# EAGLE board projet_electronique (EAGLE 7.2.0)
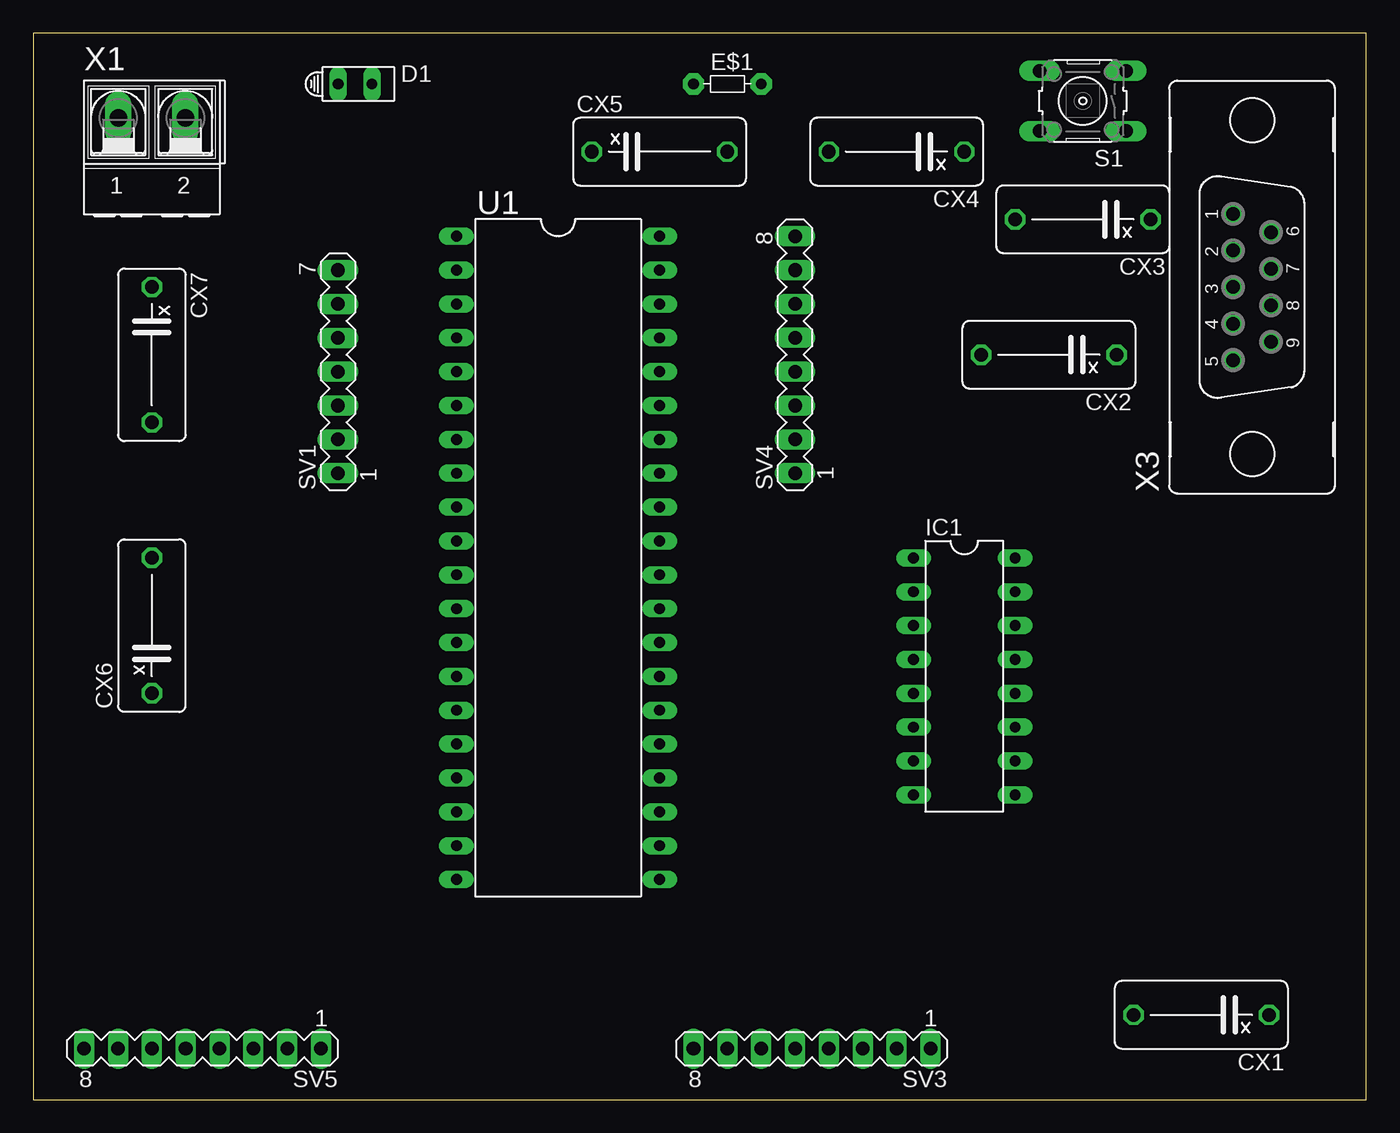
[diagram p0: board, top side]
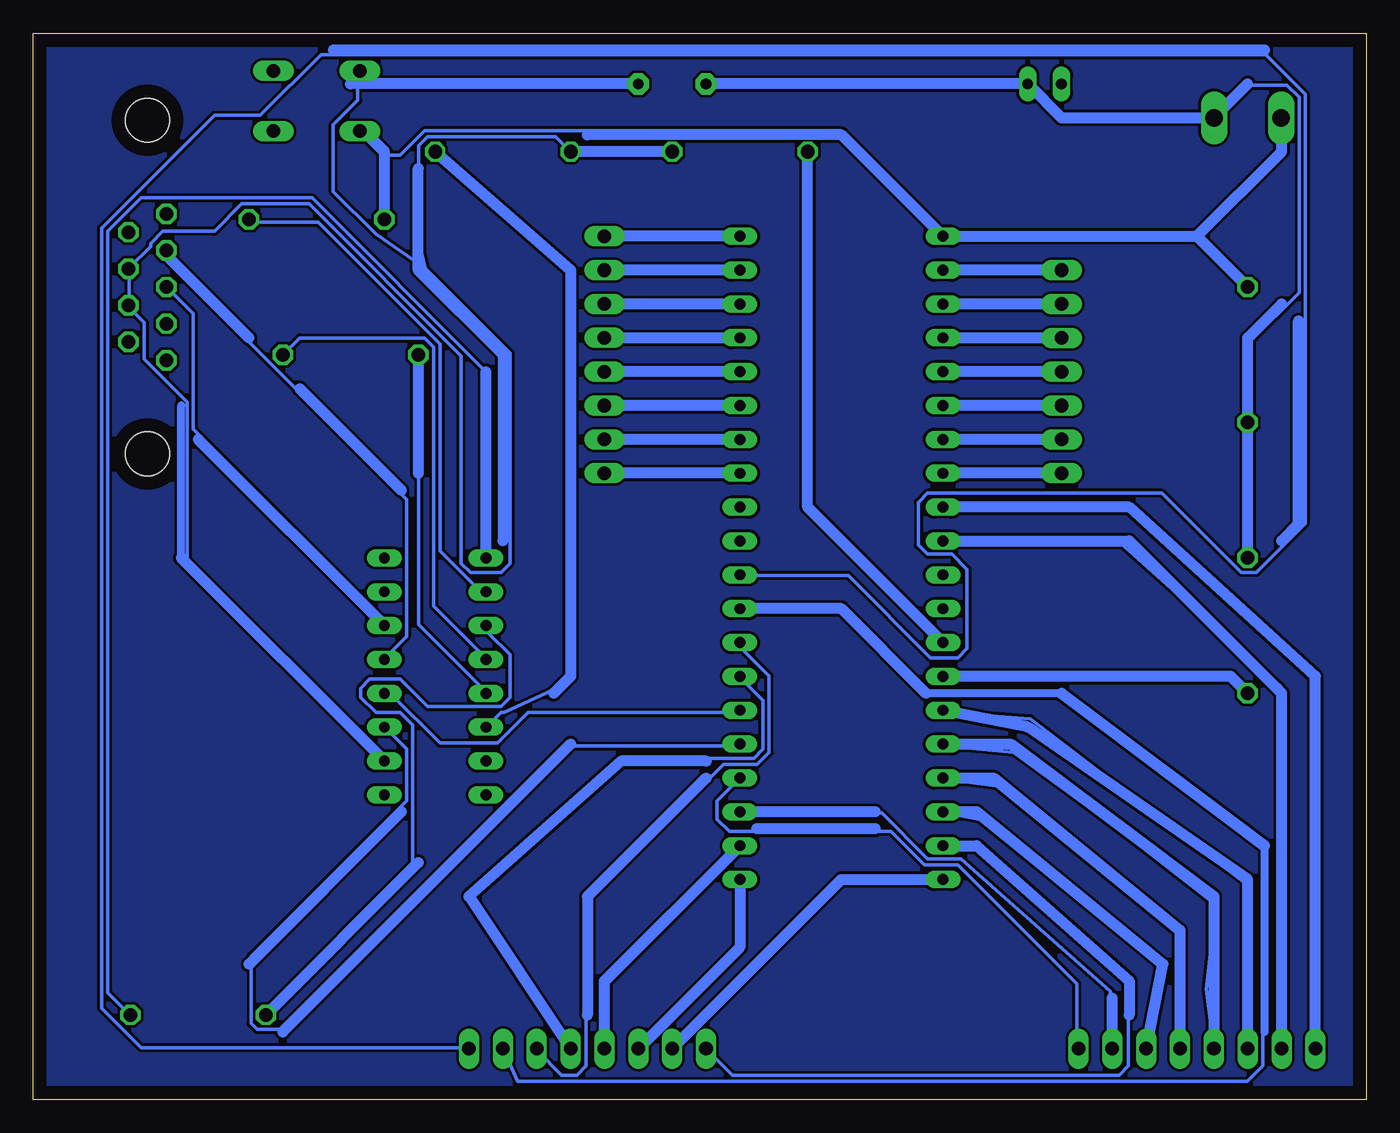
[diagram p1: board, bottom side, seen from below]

Size 100 x 80 mm. Coordinates in mm from the lower left corner, seen from the top.
Outline: 0,0 100,0 100,80 0,80 0,0
Copper layers (1*16): Top 0.035mm / dielectric 1.5mm / Bottom 0.035mm
Design rules "default": minimum track width 10mil, minimum drill 24mil, track to track 8mil, track to pad 8mil, pad to pad 8mil, via to via 8mil, smd to smd 8mil, copper to edge 40mil, drill to drill 8mil, minimum pad ring 10mil, minimum via ring 8mil, stop-mask expansion 4mil, vias tented up to drill 0mil, thermal gap 10mil

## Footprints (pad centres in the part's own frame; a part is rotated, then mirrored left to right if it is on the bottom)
XC10B5 = drill 1.016 octagon: 1 -5.08,0; 2 5.08,0
HLMP6 = drill 0.813 long: A -1.27,0; K 1.27,0
R-5 = drill 0.813 pad 1.6 octagon: 1 -2.54,0; 2 2.54,0
DIL16 = drill 0.813 long: 1 -8.89,-3.81; 2 -6.35,-3.81; 3 -3.81,-3.81; 4 -1.27,-3.81; 5 1.27,-3.81; 6 3.81,-3.81; 7 6.35,-3.81; 8 8.89,-3.81; 9 8.89,3.81; 10 6.35,3.81; 11 3.81,3.81; 12 1.27,3.81; 13 -1.27,3.81; 14 -3.81,3.81; 15 -6.35,3.81; 16 -8.89,3.81
B3F-10XX = drill 1.016 long: 1 -3.251,2.261; 2 3.251,2.261; 3 -3.251,-2.261; 4 3.251,-2.261
MA07-1 = drill 1.016 long: 1 -7.62,0; 2 -5.08,0; 3 -2.54,0; 4 0,0; 5 2.54,0; 6 5.08,0; 7 7.62,0
MA08-1 = drill 1.016 long: 1 -8.89,0; 2 -6.35,0; 3 -3.81,0; 4 -1.27,0; 5 1.27,0; 6 3.81,0; 7 6.35,0; 8 8.89,0
DIL40 = drill 0.813 long: 1 -24.13,-7.62; 2 -21.59,-7.62; 3 -19.05,-7.62; 4 -16.51,-7.62; 5 -13.97,-7.62; 6 -11.43,-7.62; 7 -8.89,-7.62; 8 -6.35,-7.62; 9 -3.81,-7.62; 10 -1.27,-7.62; 11 1.27,-7.62; 12 3.81,-7.62; 13 6.35,-7.62; 14 8.89,-7.62; 15 11.43,-7.62; 16 13.97,-7.62; 17 16.51,-7.62; 18 19.05,-7.62; 19 21.59,-7.62; 20 24.13,-7.62; 21 24.13,7.62; 22 21.59,7.62; 23 19.05,7.62; 24 16.51,7.62; 25 13.97,7.62; 26 11.43,7.62; 27 8.89,7.62; 28 6.35,7.62; 29 3.81,7.62; 30 1.27,7.62; 31 -1.27,7.62; 32 -3.81,7.62; 33 -6.35,7.62; 34 -8.89,7.62; 35 -11.43,7.62; 36 -13.97,7.62; 37 -16.51,7.62; 38 -19.05,7.62; 39 -21.59,7.62; 40 -24.13,7.62
AK500/2-H = drill 1.321 long: 1 -2.515,0; 2 2.515,0
F09V = drill 1.016 octagon: 1 5.486,1.422; 2 2.743,1.422; 3 0,1.422; 4 -2.743,1.422; 5 -5.486,1.422; 6 4.115,-1.422; 7 1.372,-1.422; 8 -1.372,-1.422; 9 -4.115,-1.422 | hole 3.302: -12.522,0; 12.522,0

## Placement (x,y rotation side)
CX1  1u  [XC10B5]  87.63,6.35 180 top
CX2  1u  [XC10B5]  76.2,55.88 180 top
CX3  1u  [XC10B5]  78.74,66.04 180 top
CX4  1u  [XC10B5]  64.77,71.12 180 top
CX5  15p  [XC10B5]  46.99,71.12 0 top
CX6  15p  [XC10B5]  8.89,35.56 90 top
CX7  680n  [XC10B5]  8.89,55.88 270 top
D1  HLMP6  [HLMP6]  24.13,76.2 0 top
E$1  [R-5]  52.07,76.2 0 top
IC1  MAX232  [DIL16]  69.85,31.75 270 top
S1  [B3F-10XX]  78.74,74.93 180 top
SV1  [MA07-1]  22.86,54.61 90 top
SV3  [MA08-1]  58.42,3.81 180 top
SV4  [MA08-1]  57.15,55.88 90 top
SV5  [MA08-1]  12.7,3.81 180 top
U1  PIC16F877P  [DIL40]  39.37,40.64 270 top
X1  [AK500/2-H]  8.89,73.66 0 top
X3  [F09V]  91.44,60.96 90 top

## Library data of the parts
CX1-CX7 = rcl
D1 = display-hp; MF: AGILENT TECHNOLOGIES; MPN: HLMP-6500; OC_FARNELL: 1652490; OC_NEWARK: 40K0088
E$1 = discrete
IC1 = maxim; MF: MAXIM; MPN: MAX232ACPE+; OC_FARNELL: 9723773; OC_NEWARK: 68K4544
S1 = switch-omron; MPN: B3F-1000; OC_FARNELL: 176432; OC_NEWARK: 36M3542
SV1 SV3-SV5 = con-lstb; OC_FARNELL: unknown; OC_NEWARK: unknown
U1 = pic16f87x
X1 = con-ptr500; OC_FARNELL: unknown; OC_NEWARK: unknown
X3 = con-subd; OC_FARNELL: unknown; OC_NEWARK: unknown

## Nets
GND: IC1.15
N$1: D1.A
N$2: CX3.2 CX7.1 S1.2 U1.1 X1.1
N$3: CX4.2 CX5.2 IC1.10 S1.4 X3.7 X3.8
N$4: CX5.1 U1.13
N$5: CX1.1 IC1.1
N$7: CX6.1 U1.14
N$8: CX1.2 IC1.3
N$9: CX2.1 IC1.4
N$10: CX2.2 IC1.5
N$11: CX3.1 IC1.2
N$12: CX4.1 IC1.6
N$13: IC1.11 U1.25
N$14: IC1.12 U1.26
N$15: SV1.7 U1.2
N$16: IC1.14 X3.3
N$17: IC1.13 X3.2
N$18: SV4.1 U1.33
N$19: SV4.2 U1.34
N$20: SV4.3 U1.35
N$21: SV4.4 U1.36
N$22: SV1.6 U1.3
N$23: SV1.5 U1.4
N$24: SV1.4 U1.5
N$25: SV1.3 U1.6
N$26: SV1.2 U1.7
N$27: SV1.1 U1.8
N$28: SV3.8 U1.19
N$29: SV3.7 U1.20
N$30: SV3.6 U1.21
N$31: SV3.5 U1.22
N$32: SV3.4 U1.27
N$33: SV3.3 U1.28
N$34: SV3.2 U1.29
N$35: SV3.1 U1.30
N$36: SV4.5 U1.37
N$37: SV4.6 U1.38
N$38: SV4.7 U1.39
N$39: SV4.8 U1.40
N$40: SV5.8 U1.9
N$41: SV5.7 U1.10
N$42: SV5.6 U1.15
N$43: SV5.5 U1.16
N$44: SV5.4 U1.17
N$45: SV5.3 U1.18
N$46: SV5.2 U1.23
N$47: SV5.1 U1.24
S$1: CX6.2 CX7.2 D1.K E$1.1 X1.2
S$2: E$1.2
VCC: IC1.16

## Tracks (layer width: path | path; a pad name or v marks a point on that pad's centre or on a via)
N$2
  Bottom 0.254: 73.84,70.87 73.84,66.06 CX3.2 | 73.84,70.87 75.44,72.47 S1.2 | 12.57,64.69 31.55,64.69 U1.1 31.77,64.92 39.55,72.69 70.64,72.69 72.47,70.87 73.84,70.87 | 12.57,64.69 8.91,61.04 CX7.1 | 12.57,64.69 6.4,70.87 6.4,73.61 X1.1
  Bottom 0.813: 12.7,64.77 U1.1 39.37,72.39 58.42,72.39 | 12.7,64.77 CX7.1 | 12.7,64.77 6.35,71.12 6.35,73.66 | CX3.2 73.66,71.12 74.93,72.39
N$3
  Bottom 0.254: IC1.10 73.84,25.6 88.47,40.23 88.47,52.35 91.67,55.55 91.67,58.29 92.81,59.44 X3.8 92.81,59.66 92.81,62.18 X3.7 92.81,62.41 91.21,64.01 91.21,64.24 90.3,65.15 86.41,65.15 84.35,67.21 79.32,67.21 67.89,55.78 67.89,40.23 67.21,39.55 64.92,39.55 64.24,40.23 64.24,56.01 70.61,62.38 | CX5.2 52.12,71.09 59.66,71.09 CX4.2 60.81,72.24 70.41,72.24 71.09,71.55 71.09,64.44 70.61,62.38 | 70.61,62.38 74.3,64.92 77.5,68.12 77.5,73.15 75.67,74.98 75.67,77.04 S1.4
  Bottom 0.61: 88.9,40.64 88.9,52.07
  Bottom 0.813: CX5.2 CX4.2 | IC1.10 88.9,40.64
N$4
  Bottom 0.254: U1.13 31.77,34.29 31.77,34.75 41.83,44.81 41.83,71.09 CX5.1
  Bottom 0.813: U1.13 41.91,44.45 CX5.1
N$5
  Bottom 0.254: IC1.1 66.06,40.69 66.06,54.63 79.1,67.67 91.9,67.67 94.41,65.15 94.41,8 92.81,6.4 CX1.1
  Bottom 0.813: IC1.1 66.04,54.61
N$7
  Bottom 0.254: U1.14 31.55,31.55 9.83,31.55 8.91,30.63 CX6.1
  Bottom 0.813: CX6.1 10.16,31.75 U1.14
N$8
  Bottom 0.254: IC1.3 65.84,35.43 65.84,34.98 64.24,33.38 64.24,30.18 64.92,29.49 70.41,29.49 72.47,31.55 74.75,31.55 75.44,30.86 75.44,30.18 74.3,29.03 72.47,29.03 71.55,28.12 71.55,17.37 82.53,6.4 CX1.2
  Bottom 0.813: CX1.2 71.12,17.78
N$9
  Bottom 0.254: CX2.1 80.01,57.15 70.64,57.15 69.95,56.46 69.95,37.03 66.06,33.15 IC1.4
N$10
  Bottom 0.254: IC1.5 66.06,30.63 71.09,35.66 71.09,55.78 CX2.2
  Bottom 0.813: CX2.2 71.12,46.99
N$11
  Bottom 0.254: IC1.2 66.06,38.18 66.52,38.18 69.49,41.15 69.49,56.69 78.64,65.84 83.67,65.84 CX3.1
N$12
  Bottom 0.254: IC1.6 65.84,28.12 64.92,29.03 64.69,29.03 59.97,31.22 59.97,62.61 69.72,71.09 CX4.1
  Bottom 0.813: CX4.1 59.69,62.23 59.69,31.75 60.96,30.48
N$13
  Bottom 0.254: IC1.11 72.01,26.29 72.01,22.4 83.67,10.74 83.67,5.71 83.21,5.26 81.38,5.26 60.12,26.52 47.09,26.52 U1.25
N$14
  Bottom 0.254: U1.26 47.09,29.03 62.87,29.03 65.15,26.75 69.49,26.75 73.15,30.4 73.61,30.4 IC1.12
N$15
  Bottom 0.254: U1.2 31.55,62.41 22.86,62.41 SV1.7
  Bottom 0.813: SV1.7 U1.2
N$16
  Bottom 0.254: IC1.14 73.84,35.66 73.84,36.12 88.01,50.29 88.01,58.98 89.84,60.81 X3.3
  Bottom 0.813: IC1.14 87.63,49.53
N$17
  Bottom 0.254: IC1.13 73.61,33.15 72.01,34.75 72.01,45.03 89.84,62.87 89.84,63.55 X3.2
N$18
  Bottom 0.254: U1.33 47.09,47.09 57.15,47.09 SV4.1
  Bottom 0.813: U1.33 SV4.1
N$19
  Bottom 0.254: U1.34 47.09,49.61 57.15,49.61 SV4.2
  Bottom 0.813: U1.34 SV4.2
N$20
  Bottom 0.254: U1.35 47.09,52.12 57.15,52.12 SV4.3
  Bottom 0.813: U1.35 SV4.3
N$21
  Bottom 0.254: U1.36 47.09,54.63 57.15,54.63 SV4.4
  Bottom 0.813: U1.36 SV4.4
N$22
  Bottom 0.254: U1.3 31.55,59.89 22.86,59.89 SV1.6
  Bottom 0.813: SV1.6 U1.3
N$23
  Bottom 0.813: SV1.5 U1.4
N$24
  Bottom 0.254: U1.5 31.55,54.63 22.86,54.63 SV1.4
  Bottom 0.813: SV1.4 U1.5
N$25
  Bottom 0.254: U1.6 31.55,52.12 22.86,52.12 SV1.3
  Bottom 0.813: SV1.3 U1.6
N$26
  Bottom 0.254: U1.7 31.55,49.61 22.86,49.61 SV1.2
  Bottom 0.813: SV1.2 U1.7
N$27
  Bottom 0.254: U1.8 31.55,47.09 22.86,47.09 SV1.1
  Bottom 0.813: SV1.1 U1.8
N$28
  Bottom 0.254: SV3.8 47.55,1.83 18.52,1.83 17.83,2.52 17.83,8.71 29.36,18.97 31.55,18.97 U1.19
  Bottom 0.813: U1.19 29.21,19.05 17.78,8.89 17.78,6.35
N$29
  Bottom 0.254: U1.20 31.77,16.46 39.32,16.46 51.89,3.89 SV3.7
  Bottom 0.813: SV3.7 39.37,16.51 U1.20
N$30
  Bottom 0.254: U1.21 47.09,16.46 47.09,11.2 54.41,3.89 SV3.6
  Bottom 0.813: U1.21 46.99,11.43 SV3.6
N$31
  Bottom 0.254: SV3.5 57.15,8.46 47.09,18.52 47.09,18.97 U1.22
  Bottom 0.813: SV3.5 57.15,8.89 U1.22
N$32
  Bottom 0.254: U1.27 46.86,31.55 45.26,29.95 45.26,26.29 45.95,25.6 56.08,25.6 67.28,15.67 59.66,3.89 SV3.4
  Bottom 0.813: 49.53,25.4 55.88,25.4 67.31,15.24 SV3.4
N$33
  Bottom 0.254: U1.28 46.86,34.29 46.86,33.83 44.81,31.77 44.81,26.06 45.72,25.15 48.23,25.15 58.52,14.86 58.52,2.52 59.21,1.83 60.35,1.83 62.18,3.66 SV3.3
N$34
  Bottom 0.254: U1.29 46.86,36.8 39.09,36.8 32.69,30.4 23.24,30.4 7.77,18.75 7.77,2.52 8.91,1.37 63.68,1.37 64.69,3.66 SV3.2
  Bottom 0.61: 7.62,5.08 7.62,19.05 | 22.86,30.48 33.02,30.48
  Bottom 0.813: 7.62,19.05 22.86,30.48 | 33.02,30.48 39.37,36.83 U1.29
N$35
  Bottom 0.254: U1.30 46.86,39.32 38.86,39.32 32.69,33.15 30.63,33.15 29.95,33.83 29.95,39.78 31.09,40.92 32.92,40.92 33.6,41.6 33.6,44.81 32.92,45.49 15.32,45.49 9.37,39.55 8.23,39.55 4.57,43.2 4.57,75.44 7.54,78.41 78.41,78.41 82.98,73.84 86.41,73.84 94.87,65.38 94.87,6.86 91.9,3.89 67.44,3.89 SV3.1
N$36
  Bottom 0.813: U1.37 SV4.5
N$37
  Bottom 0.254: U1.38 47.09,59.89 57.15,59.89 SV4.6
  Bottom 0.813: U1.38 SV4.6
N$38
  Bottom 0.254: U1.39 47.09,62.41 57.15,62.41 SV4.7
  Bottom 0.813: U1.39 SV4.7
N$39
  Bottom 0.254: U1.40 47.09,64.92 57.15,64.92 SV4.8
  Bottom 0.813: U1.40 SV4.8
N$40
  Bottom 0.254: U1.9 31.55,44.35 17.8,44.35 3.89,31.7 3.89,3.89 SV5.8
  Bottom 0.813: SV5.8 3.81,31.75 17.78,44.45 U1.9
N$41
  Bottom 0.254: U1.10 31.55,41.83 18.52,41.83 6.4,30.99 6.4,3.89 SV5.7
  Bottom 0.813: SV5.7 6.35,30.48 17.78,41.91 U1.10
N$42
  Bottom 0.254: U1.15 31.55,29.03 25.2,28.57 8.91,16.1 8.91,3.89 SV5.6
  Bottom 0.813: SV5.6 8.89,16.51 25.4,27.94 U1.15
N$43
  Bottom 0.254: U1.16 31.55,26.52 26.47,26.06 17.04,19.18 17.04,19.1 11.28,14.61 11.99,8.26 11.43,3.89 SV5.5
  Bottom 0.813: U1.16 26.67,26.67 11.43,15.24 SV5.5
N$44
  Bottom 0.254: U1.17 31.55,24 27.74,23.55 13.69,12.04 13.69,9.75 14.17,3.89 SV5.4
  Bottom 0.813: U1.17 27.94,24.13 13.97,12.7 SV5.4
N$45
  Bottom 0.254: U1.18 31.55,21.49 29.01,21.03 15.42,9.98 16.69,3.89 SV5.3
  Bottom 0.813: SV5.3 15.24,10.16 29.21,21.59 U1.18
N$46
  Bottom 0.254: U1.23 46.86,21.49 36.35,21.49 32.92,18.06 30.4,18.06 19.2,8.13 19.2,3.89 SV5.2
  Bottom 0.813: SV5.2 19.05,7.62 | 36.83,21.59 U1.23
N$47
  Bottom 0.254: U1.24 47.09,24 48.69,22.4 48.69,21.03 47.78,20.12 35.66,20.12 33.15,17.6 30.63,17.6 21.72,8.69 21.72,3.89 SV5.1
S$1
  Bottom 0.254: 25.6,76.12 D1.K 25.38,76.12 24.92,76.12 22.63,73.84 11.43,73.84 X1.2 11.2,73.84 8.91,76.12 5.94,76.12 5.03,75.21 5.03,60.55 8.69,56.9 8.69,50.98 CX7.2 8.91,50.75 8.91,40.69 CX6.2
  Bottom 0.813: E$1.1 D1.K 22.86,73.66 11.43,73.66 8.89,76.2 | CX6.2 CX7.2 8.89,57.15 6.35,59.69
S$2
  Bottom 0.813: E$1.2 76.2,76.2
S$3
  Bottom 0.813: 36.83,20.32 45.72,20.32
S$4
  Bottom 0.813: 7.62,78.74 77.47,78.74
S$5
  Bottom 0.813: 59.69,26.67 81.28,5.08
S$6
  Bottom 0.813: 83.82,10.16 72.39,21.59
S$7
  Bottom 0.813: 71.12,69.85 71.12,62.23 64.77,55.88 64.77,41.91
S$8
  Bottom 0.813: 90.17,63.5 83.82,57.15
S$9
  Bottom 0.813: 6.35,41.91 5.08,43.18 5.08,58.42
S$10
  Bottom 0.813: 80.01,53.34 72.39,45.72
S$11
  Bottom 0.813: 49.53,24.13 58.42,15.24 58.42,6.35
S$12
  pour Bottom: 0,0 0,80.01 100.33,80.01 100.33,78.74 100.33,0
